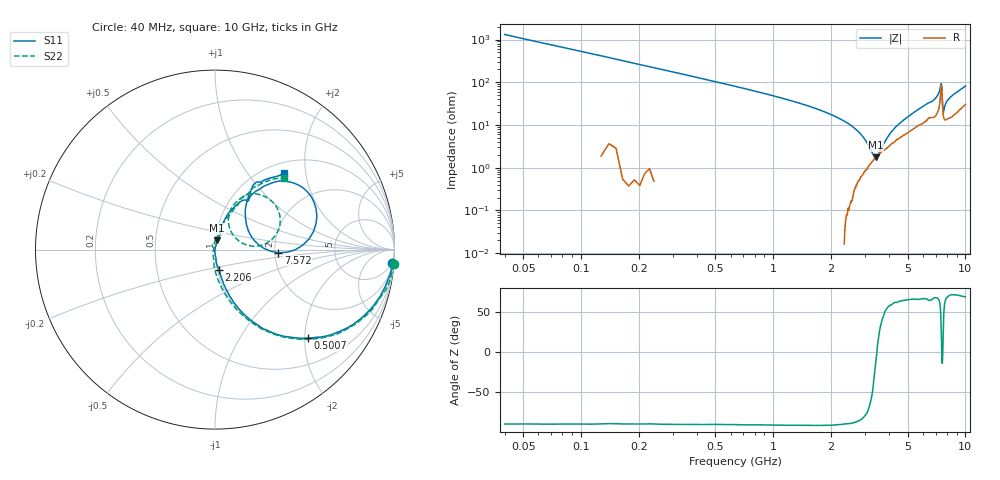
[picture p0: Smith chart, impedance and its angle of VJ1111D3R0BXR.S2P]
! VJ1111D3R0BXR
! DATE 03/04/2022  13:48
! CAPACITORS MOUNTED IN SERIES ON 25 MIL THICK MICROSTRIP SUBSTRATE
# GHz  S  MA  R  50.00
!  FREQ  S11M  S11A  S21M  S21A  S12M  S12A  S22M  S22A
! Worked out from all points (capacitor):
!   801 points, 40 MHz to 10 GHz, reference 50 ohm
!   read as one part in series: C = 3.02 pF near 89.8 MHz
!   lowest |Z| = 1.77 ohm at 3.414 GHz (marker M1)
!   series resonance near 3.465 GHz, so ESL is about 700 pH
!   S11 on the Smith chart (normalised r, x): 40 MHz: 4, -26; 500.7 MHz: 1.02, -2.08; 2.206 GHz: 1.02, -0.23; 7.572 GHz: 2.09, -0.08; 10 GHz: 1.20, +1.53
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0.04  0.9899 -4.3  0.0757 85.5  0.07561 85.7  1 -4.7
0.2143  0.9228 -21.7  0.3787 68.0  0.3789 68.6  0.9303 -21.9
0.50065  0.7165 -43.6  0.7007 46.6  0.7029 46.8  0.7187 -44.1
0.9862  0.4344 -63.5  0.9067 27.2  0.9107 27.1  0.4312 -64.9
1.7083  0.2075 -75.3  0.9787 14.5  0.9841 14.4  0.2064 -80.8
2.2063  0.1149 -78.9  0.9846 9.8  0.9901 9.6  0.1128 -90.5
2.76655  0.03193 -86.5  0.9792 6.3  0.9845 6.2  0.03541 -106.7
2.86615  0.01629 -92.4  0.9775 5.9  0.9827 5.7  0.02222 -117.3
2.96575  0.001279 -88.6  0.9766 5.4  0.9818 5.2  0.01266 -140.1
3.11515  0.02014 74.3  0.9778 4.7  0.9826 4.6  0.00931 128.5
3.36415  0.04742 77.3  0.9705 3.4  0.9758 3.2  0.03232 97.3
3.41395  0.05376 76.8  0.97 3.3  0.9747 3.1  0.03825 95.5
3.775  0.09075 67.9  0.9709 1.6  0.9752 1.5  0.07439 79.0
5.02  0.1934 70.9  0.9037 -4.5  0.908 -4.7  0.1622 71.7
6.6883  0.3376 56.0  0.8046 -12.0  0.8084 -12.2  0.3072 63.2
7.3606  0.5588 42.5  0.6627 -18.8  0.6663 -19.0  0.4036 47.8
7.4851  0.5975 18.2  0.5218 -8.7  0.5242 -8.8  0.4091 28.2
7.57225  0.3537 -2.8  0.6784 8.6  0.6815 8.4  0.2496 4.9
7.6594  0.2139 30.4  0.8247 0.1  0.8282 -0.2  0.1328 46.6
7.8835  0.3287 56.7  0.8258 -10.2  0.8296 -10.4  0.2693 67.5
8.34415  0.4271 59.1  0.7857 -15.7  0.7901 -15.8  0.3599 59.6
10  0.5753 47.9  0.6309 -24.2  0.634 -24.4  0.5506 46.1
